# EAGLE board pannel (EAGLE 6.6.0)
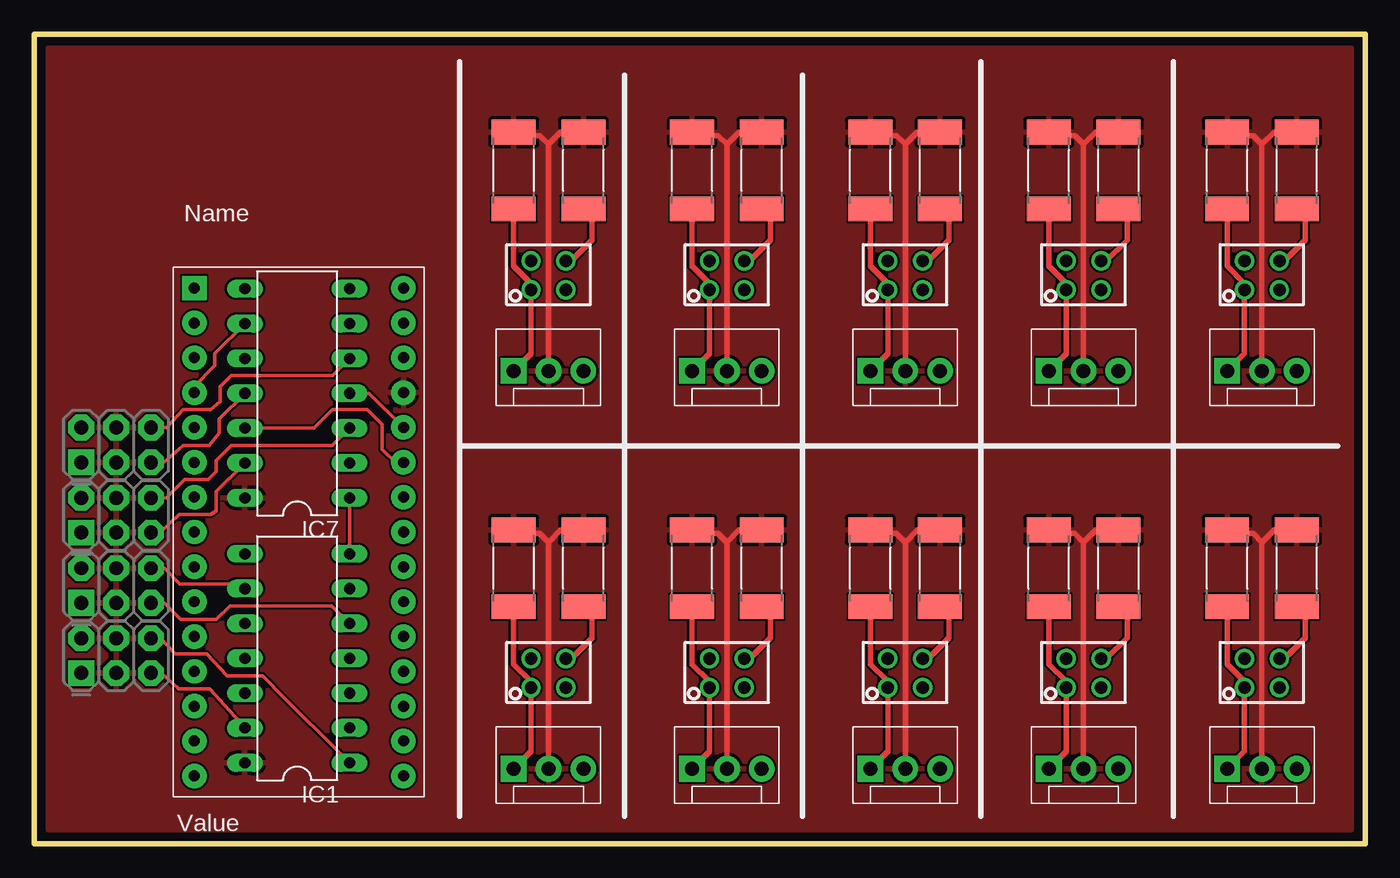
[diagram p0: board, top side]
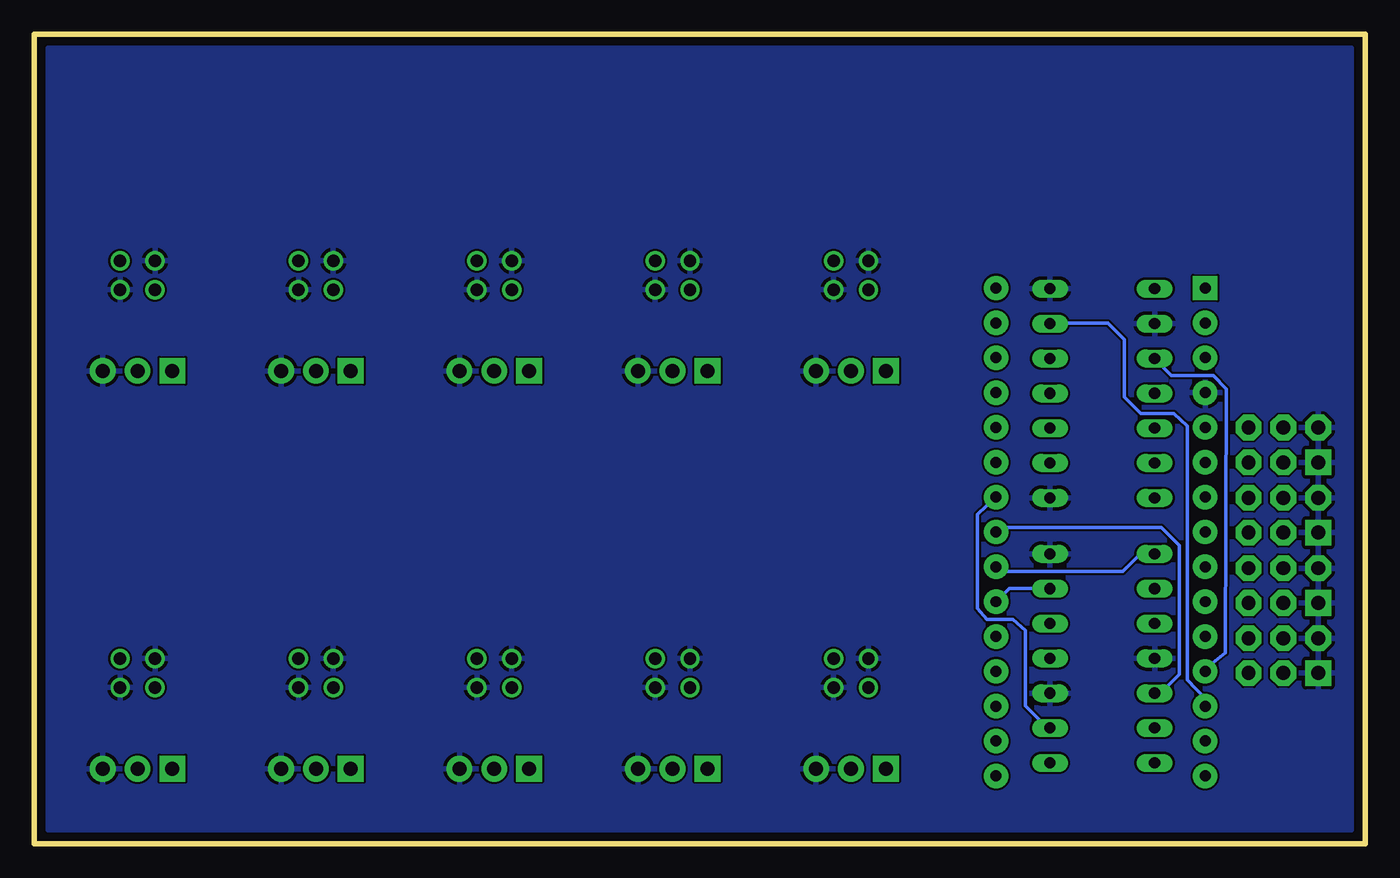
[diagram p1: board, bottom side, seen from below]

Size 97 x 59 mm. Coordinates in mm from the lower left corner, seen from the top.
Outline: 0,59 0,0 97,0 97,59 0,59
Copper layers (1*16): Top 0.035mm / dielectric 1.5mm / Bottom 0.035mm
Design rules "SeeedStudio_2layer_DRU_no_angle_20140221": minimum track width 6mil, minimum drill 12mil, track to track 6mil, track to pad 6mil, pad to pad 6mil, via to via 6mil, smd to smd 0mil, copper to edge 10mil, drill to drill 10mil, minimum pad ring 10mil, minimum via ring 6mil, stop-mask expansion 2mil, vias tented up to drill 100mil, thermal gap 10mil

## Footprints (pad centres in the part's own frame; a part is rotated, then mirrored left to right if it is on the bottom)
DIL14 = drill 0.813 long: 1 -7.62,-3.81; 2 -5.08,-3.81; 3 -2.54,-3.81; 4 0,-3.81; 5 2.54,-3.81; 6 5.08,-3.81; 7 7.62,-3.81; 8 7.62,3.81; 9 5.08,3.81; 10 2.54,3.81; 11 0,3.81; 12 -2.54,3.81; 13 -5.08,3.81; 14 -7.62,3.81
MOLEX-1X3 = drill 1.016 pad 1.88 square: 1 0,0 | drill 1.016 pad 1.88: 2 2.54,0; 3 5.08,0
2X3-NS = drill 1.016 pad 1.88 square: 1 -2.54,-1.27 | drill 1.016 pad 1.88 octagon: 2 -2.54,1.27; 3 0,-1.27; 4 0,1.27; 5 2.54,-1.27; 6 2.54,1.27
R2512 = smd 1.8 x 3.2: 1 -2.8,0; 2 2.8,0
QRD1114 = drill 0.9: 1 -1.067,1.27; 2 -1.067,-1.27; 3 1.041,-1.27; 4 1.041,1.27
PDIP-32 = drill 0.8 pad 1.778: 3V3 15.24,-35.56; +5V 15.24,-10.16; A0 15.24,-12.7; A1 15.24,-15.24; A2 15.24,-17.78; A3 15.24,-20.32; A4 15.24,-22.86; A5 15.24,-25.4; A6 15.24,-27.94; A7 15.24,-30.48; AREF 15.24,-33.02; D0/RX 0,-5.08; D2 0,-12.7; D3 0,-15.24; D4 0,-17.78; D5 0,-20.32; D6 0,-22.86; D7 0,-25.4; D8 0,-27.94; D9 0,-30.48; D10 0,-33.02; D11 0,-35.56; D12 0,-38.1; D13 15.24,-38.1; GND 0,-10.16; GND1 15.24,-5.08; RESET 0,-7.62; RESET1 15.24,-7.62; VIN 15.24,-2.54 | drill 0.8 pad 1.778 square: D1/TX 0,-2.54

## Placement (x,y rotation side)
IC1  7414N  [DIL14]  19.16,13.51 90 top
IC7  7414N  [DIL14]  19.16,32.83 90 top
JP1  [MOLEX-1X3]  34.94,5.46 0 top
JP2  [2X3-NS]  5.96,18.81 0 top
JP3  [2X3-NS]  5.96,13.71 0 top
JP4  [2X3-NS]  5.96,23.94 0 top
JP5  [MOLEX-1X3]  47.94,5.46 0 top
JP6  [MOLEX-1X3]  34.94,34.47 0 top
JP7  [MOLEX-1X3]  86.94,5.46 0 top
JP8  [MOLEX-1X3]  47.94,34.47 0 top
JP9  [MOLEX-1X3]  86.94,34.47 0 top
JP10  [MOLEX-1X3]  60.94,5.46 0 top
JP11  [MOLEX-1X3]  73.94,5.46 0 top
JP12  [2X3-NS]  5.96,29.07 0 top
JP13  [MOLEX-1X3]  60.94,34.47 0 top
JP14  [MOLEX-1X3]  73.94,34.47 0 top
R1  330  [R2512]  40.02,20.07 90 top
R2  10K  [R2512]  34.94,20.07 90 top
R3  330  [R2512]  53.02,20.07 90 top
R4  10K  [R2512]  47.94,20.07 90 top
R5  330  [R2512]  40.02,49.07 90 top
R6  10K  [R2512]  34.94,49.07 90 top
R7  330  [R2512]  92.02,20.07 90 top
R8  10K  [R2512]  86.94,20.07 90 top
R9  330  [R2512]  53.02,49.07 90 top
R10  10K  [R2512]  47.94,49.07 90 top
R11  330  [R2512]  92.02,49.07 90 top
R12  10K  [R2512]  86.94,49.07 90 top
R13  330  [R2512]  66.02,20.07 90 top
R14  10K  [R2512]  60.94,20.07 90 top
R15  330  [R2512]  79.02,20.07 90 top
R16  10K  [R2512]  73.94,20.07 90 top
R17  330  [R2512]  66.02,49.07 90 top
R18  10K  [R2512]  60.94,49.07 90 top
R19  330  [R2512]  79.02,49.07 90 top
R20  10K  [R2512]  73.94,49.07 90 top
U$1  QRD1114  [QRD1114]  37.48,12.45 90 top
U$2  ARDUINONANO  [PDIP-32]  11.66,43.04 0 top
U$3  QRD1114  [QRD1114]  50.48,12.45 90 top
U$4  QRD1114  [QRD1114]  37.48,41.45 90 top
U$5  QRD1114  [QRD1114]  89.47,12.45 90 top
U$6  QRD1114  [QRD1114]  50.48,41.45 90 top
U$7  QRD1114  [QRD1114]  89.47,41.45 90 top
U$8  QRD1114  [QRD1114]  63.47,12.45 90 top
U$9  QRD1114  [QRD1114]  76.47,12.45 90 top
U$10  QRD1114  [QRD1114]  63.47,41.45 90 top
U$11  QRD1114  [QRD1114]  76.47,41.45 90 top

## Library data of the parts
IC1 IC7 = 74xx-us
JP1-JP14 = SparkFun-Connectors
R1-R20 = resistor
U$1 U$3-U$11 = SparkFun-Sensors
U$2 = jet-lib

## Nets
5V: IC1.14 IC7.14 JP1.2 JP2.3 JP2.4 JP3.3 JP3.4 JP4.3 JP4.4 JP5.2 JP6.2 JP7.2 JP8.2 JP9.2 JP10.2 JP11.2 JP12.3 JP12.4 JP13.2 JP14.2 R1.2 R2.2 R3.2 R4.2 R5.2 R6.2 R7.2 R8.2 R9.2 R10.2 R11.2 R12.2 R13.2 R14.2 R15.2 R16.2 R17.2 R18.2 R19.2 R20.2 U$2.+5V
GND: IC1.3 IC1.7 IC1.11 IC7.1 IC7.7 IC7.9 JP1.3 JP2.1 JP2.2 JP3.1 JP3.2 JP4.1 JP4.2 JP5.3 JP6.3 JP7.3 JP8.3 JP9.3 JP10.3 JP11.3 JP12.1 JP12.2 JP13.3 JP14.3 U$1.2 U$1.4 U$2.GND U$3.2 U$3.4 U$4.2 U$4.4 U$5.2 U$5.4 U$6.2 U$6.4 U$7.2 U$7.4 U$8.2 U$8.4 U$9.2 U$9.4 U$10.2 U$10.4 U$11.2 U$11.4
N$1: R1.1 U$1.3
N$2: R3.1 U$3.3
N$3: R5.1 U$4.3
N$4: R7.1 U$5.3
N$5: R9.1 U$6.3
N$6: R11.1 U$7.3
N$7: R13.1 U$8.3
N$8: R15.1 U$9.3
N$9: R17.1 U$10.3
N$10: R19.1 U$11.3
RPM1: IC7.4 U$2.A0
RPM2: IC7.12 U$2.A1
RPM3: IC1.2 U$2.A2
RPM4: IC1.12 U$2.A3
RPM5: IC1.8 U$2.A4
RPM6: IC1.6 U$2.A5
RPM7: IC7.10 U$2.D9
RPM8: IC7.6 U$2.D10
SENSE1: IC7.3 JP4.6
SENSE2: IC7.13 JP4.5
SENSE3: IC1.1 JP3.6
SENSE4: IC1.13 JP3.5
SENSE5: IC1.9 JP2.6
SENSE6: IC1.5 JP2.5
SENSE7: IC7.11 JP12.5
SENSE8: IC7.5 JP12.6
SIGNAL: JP1.1 R2.1 U$1.1
SIGNAL1: JP5.1 R4.1 U$3.1
SIGNAL2: JP6.1 R6.1 U$4.1
SIGNAL3: JP7.1 R8.1 U$5.1
SIGNAL4: JP8.1 R10.1 U$6.1
SIGNAL5: JP9.1 R12.1 U$7.1
SIGNAL6: JP10.1 R14.1 U$8.1
SIGNAL7: JP11.1 R16.1 U$9.1
SIGNAL8: JP13.1 R18.1 U$10.1
SIGNAL9: JP14.1 R20.1 U$11.1

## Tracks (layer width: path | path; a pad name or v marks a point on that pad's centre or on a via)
5V
  Top 0.406: JP1.2 37.48,21.98 | R2.2 35.2,22.61 36.84,22.61 37.48,21.98 | R1.2 38.37,22.87 37.48,21.98 | JP13.2 63.47,50.98 | R18.2 61.2,51.61 62.84,51.61 63.47,50.98 | R17.2 64.37,51.87 63.47,50.98 | JP6.2 37.48,50.98 | R6.2 35.2,51.61 36.84,51.61 37.48,50.98 | R5.2 38.37,51.87 37.48,50.98 | JP8.2 50.48,50.98 | R10.2 48.2,51.61 49.84,51.61 50.48,50.98 | R9.2 51.37,51.87 50.48,50.98 | JP14.2 76.47,50.98 | R20.2 74.19,51.61 75.84,51.61 76.47,50.98 | R19.2 77.37,51.87 76.47,50.98 | JP9.2 89.47,50.98 | R12.2 87.19,51.61 88.84,51.61 89.47,50.98 | R11.2 90.37,51.87 89.47,50.98 | JP7.2 89.47,21.98 | R8.2 87.19,22.61 88.84,22.61 89.47,21.98 | R7.2 90.37,22.87 89.47,21.98 | JP11.2 76.47,21.98 | R16.2 74.19,22.61 75.84,22.61 76.47,21.98 | R15.2 77.37,22.87 76.47,21.98 | JP10.2 63.47,21.98 | R14.2 61.2,22.61 62.84,22.61 63.47,21.98 | R13.2 64.37,22.87 63.47,21.98 | JP5.2 50.48,21.98 | R4.2 48.2,22.61 49.84,22.61 50.48,21.98 | R3.2 51.37,22.87 50.48,21.98
  pour Top: 1,58 1,1 96,1 96,57 96,58
GND
  Top 0.254: IC1.7 IC7.1 | U$2.GND 11.66,33.34 13.16,34.84 13.16,35.72 IC7.9
  pour Bottom: 1,57 1,1 96,1 96,58 1,58
N$1
  Top 0.406: U$1.3 39.15,13.49 40.65,14.99 40.65,16.63 R1.1
N$2
  Top 0.406: U$3.3 52.15,13.49 53.65,14.99 53.65,16.63 R3.1
N$3
  Top 0.406: U$4.3 39.15,42.49 40.65,43.99 40.65,45.63 R5.1
N$4
  Top 0.406: U$5.3 91.15,13.49 92.65,14.99 92.65,16.63 R7.1
N$5
  Top 0.406: U$6.3 52.15,42.49 53.65,43.99 53.65,45.63 R9.1
N$6
  Top 0.406: U$7.3 91.15,42.49 92.65,43.99 92.65,45.63 R11.1
N$7
  Top 0.406: U$8.3 65.15,13.49 66.65,14.99 66.65,16.63 R13.1
N$8
  Top 0.406: U$9.3 78.15,13.49 79.65,14.99 79.65,16.63 R15.1
N$9
  Top 0.406: U$10.3 65.15,42.49 66.65,43.99 66.65,45.63 R17.1
N$10
  Top 0.406: U$11.3 78.15,42.49 79.65,43.99 79.65,45.63 R19.1
RPM1
  Top 0.254: IC7.4 24.41,32.83 U$2.A0
RPM2
  Top 0.254: IC7.12 20.41,30.29 21.76,31.64 24.26,31.64 25.36,30.54 25.36,28.74 26.36,27.74 26.84,27.74 U$2.A1
RPM3
  Bottom 0.254: IC1.2 23.15,8.43 24.76,10.04 24.76,15.54 25.66,16.34 27.56,16.34 28.26,17.14 28.26,24 U$2.A2
RPM4
  Bottom 0.254: IC1.12 14.93,10.97 13.56,12.34 13.56,21.74 14.86,23.04 26.58,23.04 U$2.A3
RPM5
  Bottom 0.254: IC1.8 16.37,21.13 17.66,19.84 26.36,19.84 U$2.A4
RPM6
  Bottom 0.254: IC1.6 25.95,18.59 U$2.A5
RPM7
  Bottom 0.254: U$2.D9 11.66,12.74 10.21,13.89 10.11,33.14 11.06,34.14 14.12,34.14 IC7.10
RPM8
  Bottom 0.254: U$2.D10 11.66,10.54 12.96,11.94 12.96,30.44 13.96,31.34 16.36,31.34 17.56,32.54 17.56,36.74 18.76,37.94 22.94,37.94 IC7.6
SENSE1
  Top 0.254: JP4.6 9.63,25.21 10.96,26.54 12.66,26.54 13.26,27.14 13.26,27.94 14.36,29.04 21.72,29.04 IC7.3
SENSE2
  Top 0.254: JP4.5 9.19,22.67 10.56,23.99 12.86,23.99 13.26,24.24 13.26,25.66 IC7.13
SENSE3
  Top 0.254: JP3.6 9.22,14.97 10.26,13.84 12.56,13.84 14.06,12.24 16.66,12.24 17.46,11.44 17.46,11.4 IC1.1
SENSE4
  Top 0.254: JP3.5 9.27,12.44 10.51,11.29 12.79,11.29 IC1.13
SENSE5
  Top 0.254: JP2.6 9.52,20.08 10.61,18.94 15.1,18.94 IC1.9
SENSE6
  Top 0.254: JP2.5 9.46,17.54 10.66,16.34 13.26,16.34 14.26,17.34 21.68,17.34 IC1.5
SENSE7
  Top 0.254: JP12.5 9.42,27.8 10.86,29.04 12.76,29.04 13.46,29.94 13.46,30.94 IC7.11
SENSE8
  Top 0.254: JP12.6 9.66,30.34 10.86,31.64 12.86,31.64 13.56,32.24 13.56,33.34 14.36,34.14 21.74,34.14 IC7.5
SIGNAL
  Top 0.406: JP1.1 36.2,6.73 U$1.1 36.2,11.82 34.94,13.09 R2.1
SIGNAL1
  Top 0.406: JP5.1 49.2,6.73 U$3.1 49.2,11.82 47.94,13.09 R4.1
SIGNAL2
  Top 0.406: JP6.1 36.2,35.73 U$4.1 36.2,40.81 34.94,42.09 R6.1
SIGNAL3
  Top 0.406: JP7.1 88.2,6.73 U$5.1 88.2,11.82 86.94,13.09 R8.1
SIGNAL4
  Top 0.406: JP8.1 49.2,35.73 U$6.1 49.2,40.81 47.94,42.09 R10.1
SIGNAL5
  Top 0.406: JP9.1 88.2,35.73 U$7.1 88.2,40.81 86.94,42.09 R12.1
SIGNAL6
  Top 0.406: JP10.1 62.2,6.73 U$8.1 62.2,11.82 60.94,13.09 R14.1
SIGNAL7
  Top 0.406: JP11.1 75.2,6.73 U$9.1 75.2,11.82 73.94,13.09 R16.1
SIGNAL8
  Top 0.406: JP13.1 62.2,35.73 U$10.1 62.2,40.81 60.94,42.09 R18.1
SIGNAL9
  Top 0.406: JP14.1 75.2,35.73 U$11.1 75.2,40.81 73.94,42.09 R20.1

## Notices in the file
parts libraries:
SparkFun-Sensors: Licensing: Creative Commons ShareAlike 4.0 International - https://creativecommons.org/licenses/by-sa/4.0
